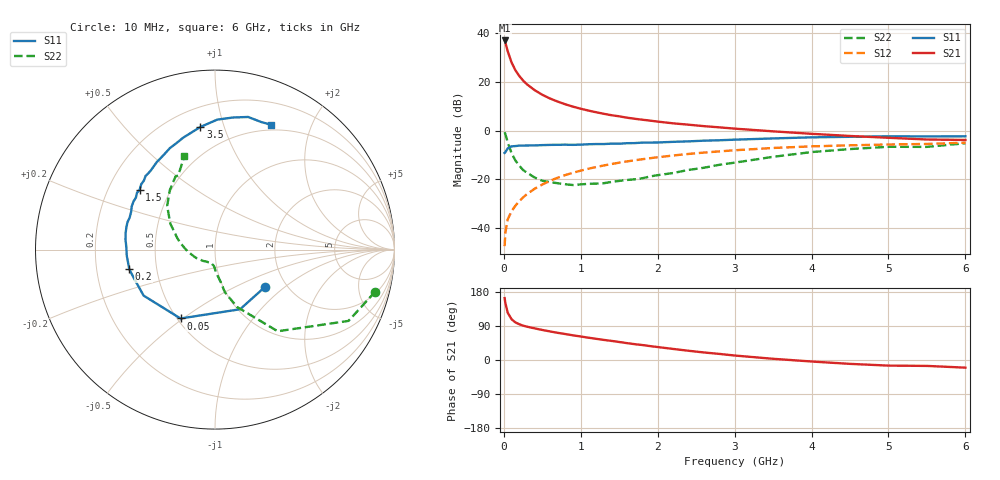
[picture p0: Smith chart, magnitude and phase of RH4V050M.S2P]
! SIEMENS Small Signal Semiconductors
! BFR106
! Si NPN RF Bipolar Junction Transistor in SOT23
! VCE = 4 V  IC = 50 mA
! Common Emitter S-Parameters:  August  1996
# GHz  S  MA  R  50
!  f  S11  S21  S12  S22
! GHz  MAG  ANG  MAG  ANG  MAG  ANG  MAG  ANG
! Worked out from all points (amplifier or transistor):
!   36 points, 10 MHz to 6 GHz, reference 50 ohm
!   highest |S21| = 37.0 dB at 10 MHz (marker M1)
!   |S21| within 3 dB of that: start of sweep to 37.94 MHz
!   unconditionally stable (mu >= 1): 243.4 MHz to 2.317 GHz
!   at 250 MHz: K = 1.01, MAG = 23.5 dB, |S12| = -27.5 dB
!   at 1.4 GHz: K = 1.05, MAG = 8.6 dB, |S12| = -13.8 dB
!   at 6 GHz: K = 0.99, MSG = 0.6 dB, |S12| = -5.0 dB
!   S11 on the Smith chart (normalised r, x): 10 MHz: 1.55, -0.74; 50 MHz: 0.52, -0.49; 200 MHz: 0.35, -0.10; 1.5 GHz: 0.34, +0.31; 3.5 GHz: 0.32, +0.84; 6 GHz: 0.44, +1.45
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0.01  0.3471 -37.1  71 163.3  0.0042 80.7  0.9228 -14.7
0.02  0.3606 -67.2  63.9 150.2  0.008 72.5  0.8434 -28.1
0.05  0.4292 -116.6  42.78 124.9  0.0149 60.3  0.5736 -52.5
0.1  0.4732 -147.2  25.16 107.6  0.0219 61.4  0.3422 -69.0
0.15  0.4794 -160.8  17.36 99.2  0.0285 64.5  0.2434 -77.0
0.2  0.4898 -167.1  13.26 94.4  0.0352 67.4  0.1898 -79.5
0.25  0.49 -172.4  10.66 90.7  0.0422 68.9  0.1543 -83.2
0.3  0.4926 -175.8  8.928 88.0  0.0492 70.3  0.1362 -86.1
0.4  0.4946 178.1  6.765 83.5  0.0635 71.6  0.1083 -90.2
0.5  0.5015 173.7  5.43 79.3  0.0777 71.7  0.0927 -93.2
0.6  0.5065 169.7  4.552 75.4  0.0925 71.2  0.0867 -96.7
0.7  0.5092 165.7  3.932 71.7  0.1072 70.4  0.0827 -101.5
0.9  0.5078 159.5  3.089 65.1  0.1358 68.3  0.0758 -109.2
1.1  0.5226 152.6  2.569 58.9  0.1641 65.9  0.0803 -119.1
1.5  0.5354 141.7  1.96 47.5  0.2185 60.1  0.0922 -137.2
1.7  0.5516 136.0  1.746 41.8  0.2442 57.2  0.0994 -147.5
2.2  0.5852 123.8  1.406 29.2  0.3069 49.6  0.1338 -168.3
3  0.6489 105.7  1.094 11.8  0.3929 37.1  0.2186 163.3
3.5  0.688 96.8  0.962 3.2  0.438 29.6  0.2882 149.8
4.5  0.7429 82.2  0.773 -10.2  0.4963 15.0  0.4158 127.3
5.5  0.756 70.0  0.654 -15.6  0.5297 5.5  0.461 116.4
6  0.7628 65.9  0.64 -20.2  0.5627 -1.6  0.5479 108.1
